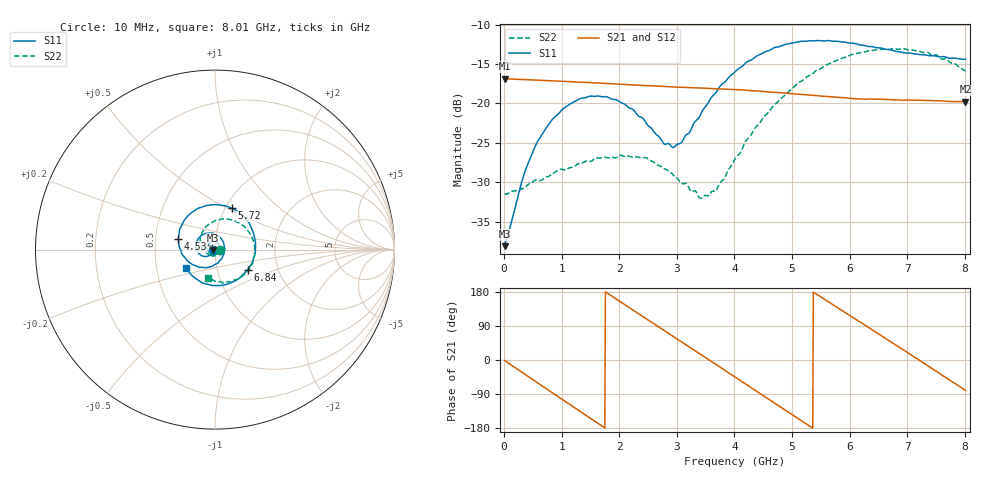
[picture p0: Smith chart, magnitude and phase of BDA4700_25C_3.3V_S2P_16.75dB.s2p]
!Agilent Technologies,E5071B,MY42404982,A.09.10
!Date: Mon Oct 20 18:10:04 2025
!Data & Calibration Information:
!Freq	S11:SOLT2(ON)	S21:SOLT2(ON)	S12:SOLT2(ON)	S22:SOLT2(ON)
# Hz S RI R 50
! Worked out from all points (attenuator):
!   801 points, 10 MHz to 8.01 GHz, reference 50 ohm
!   highest |S21| = -16.84 dB at 10 MHz (marker M1); lowest = -19.8 dB at 8.01 GHz (marker M2)
!   lowest |S11| = -38.1 dB at 10 MHz (marker M3), VSWR 1.03, Z = 48.8 - j0.156 ohm
!   |S11| at or under -10 dB: start of sweep to end of sweep
!   |S22| runs from -32.0 to -13.0 dB; largest |S21 - S12| = 0.0017
!   S11 on the Smith chart (normalised r, x): 10 MHz: 0.98, -0.00; 4.53 GHz: 0.66, +0.08; 5.72 GHz: 1.07, +0.53; 6.84 GHz: 1.40, -0.33; 8.01 GHz: 0.71, -0.15
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1e7  -0.0123 -0.0016  0.1439 -0.00316  0.1438 -0.00322  0.0266 -0.000832
3.5e8  -0.0234 -0.0268  0.114 -0.0843  0.1138 -0.0843  0.0226 -0.0182
5.7e8  -0.0418 -0.0377  0.0724 -0.1206  0.0722 -0.1206  0.0147 -0.0291
8.7e8  -0.0739 -0.034  0.000747 -0.139  0.000781 -0.1391  -0.00678 -0.0357
1.35e9  -0.1067 0.0168  -0.1023 -0.0903  -0.1022 -0.0904  -0.038 -0.0174
1.97e9  -0.0544 0.0894  -0.1237 0.0481  -0.1238 0.0481  -0.0337 0.0309
2.45e9  0.0217 0.0737  -0.0459 0.1214  -0.0459 0.1215  0.000601 0.0454
2.68e9  0.0472 0.0403  0.00508 0.1286  0.00484 0.1286  0.0169 0.0367
2.96e9  0.0513 -0.0127  0.0637 0.11  0.0637 0.1099  0.0285 0.0195
3.09e9  0.0434 -0.0369  0.0868 0.0924  0.086 0.0928  0.0299 0.00856
3.42e9  -0.00492 -0.086  0.1215 0.0306  0.1215 0.0306  0.0192 -0.0161
3.69e9  -0.0653 -0.0993  0.1208 -0.0273  0.1209 -0.0277  -0.00165 -0.0282
4.01e9  -0.1416 -0.0721  0.087 -0.0865  0.087 -0.0862  -0.0352 -0.027
4.53e9  -0.2044 0.059  -0.0146 -0.1183  -0.0145 -0.1183  -0.0796 0.0258
4.92e9  -0.1623 0.1755  -0.0836 -0.0807  -0.0832 -0.0812  -0.0735 0.0913
5.35e9  -0.0373 0.247  -0.1127 -0.00231  -0.1127 -0.00303  -0.0137 0.1526
5.72e9  0.0925 0.2307  -0.0899 0.0633  -0.0898 0.0634  0.0708 0.1697
6.22e9  0.2112 0.1011  -0.0122 0.1057  -0.0106 0.1062  0.1814 0.1078
6.68e9  0.2104 -0.0623  0.0662 0.0826  0.0664 0.0825  0.2205 -0.00896
6.84e9  0.1811 -0.113  0.0854 0.0616  0.0857 0.0608  0.214 -0.0525
7.43e9  -0.000942 -0.2007  0.0965 -0.0399  0.0965 -0.0401  0.1109 -0.1692
8.01e9  -0.1602 -0.1039  0.0174 -0.1011  0.0177 -0.1011  -0.0365 -0.1558
